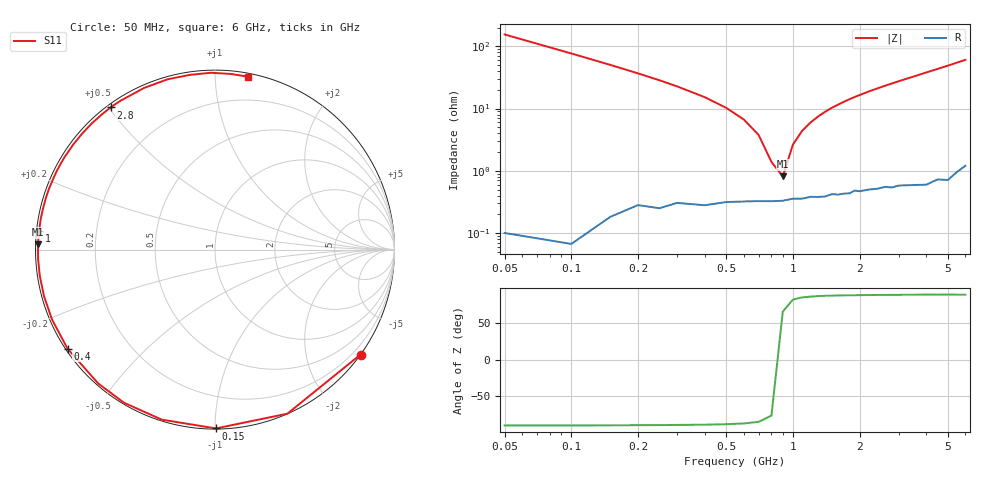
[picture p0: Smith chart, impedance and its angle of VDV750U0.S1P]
! Infineon Technologies  Discrete & RF Semiconductors
! BBY 55-03
! Si Tuning Diode in SOD323
! VR = 0.75 V
! S-Parameters:  June  1999
# GHz  S  MA  R  50
!  f  S11
! GHz  MAG  ANG
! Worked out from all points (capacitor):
!   34 points, 50 MHz to 6 GHz, reference 50 ohm
!   read as one part to ground: C = 20.5 pF near 50 MHz
!   lowest |Z| = 812 mohm at 900 MHz (marker M1)
!   series resonance near 864.6 MHz, so ESL is about 1.7 nH
!   S11 on the Smith chart (normalised r, x): 50 MHz: 0.00, -3.10; 150 MHz: 0.00, -1.01; 400 MHz: 0.01, -0.30; 1 GHz: 0.01, +0.05; 2.8 GHz: 0.01, +0.51; 6 GHz: 0.02, +1.21
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0.05  0.9996 -35.8
0.1  0.9992 -66.2
0.15  0.9964 -89.7
0.2  0.9927 -107.4
0.25  0.9924 -120.7
0.3  0.9899 -131.1
0.4  0.9898 -146.1
0.5  0.988 -156.8
0.6  0.9874 -164.8
0.7  0.9871 -171.4
0.8  0.9871 -176.9
0.9  0.9868 178.3
1  0.9858 174.0
1.1  0.9859 170.0
1.3  0.9852 163.0
1.6  0.9844 153.9
1.8  0.984 148.4
2  0.9832 143.5
2.2  0.9826 138.7
2.4  0.9826 134.4
2.8  0.9829 126.3
3  0.9823 122.4
3.5  0.9835 113.7
4  0.9849 105.5
4.5  0.9835 98.1
5  0.9855 91.3
5.5  0.9827 84.8
6  0.9806 79.1
